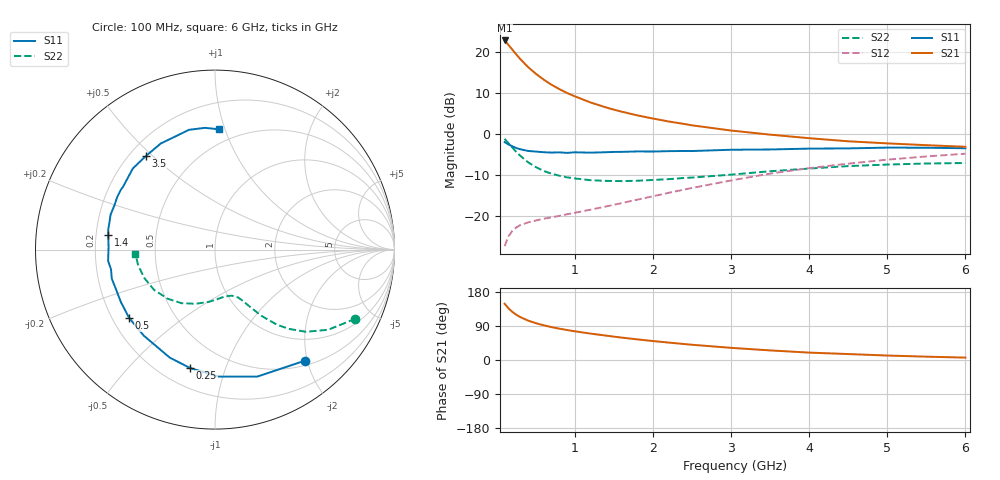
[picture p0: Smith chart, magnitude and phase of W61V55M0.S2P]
! SIEMENS Small Signal Semiconductors
! BFR193W
! Si NPN RF Bipolar Junction Transistor in SOT323
! VCE = 1.5 V  IC = 5 mA
! Common Emitter S-Parameters:  September  1992
# GHz  S  MA  R  50
!  f  S11  S21  S12  S22
! GHz  MAG  ANG  MAG  ANG  MAG  ANG  MAG  ANG
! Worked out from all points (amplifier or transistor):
!   28 points, 100 MHz to 6 GHz, reference 50 ohm
!   highest |S21| = 22.8 dB at 100 MHz (marker M1)
!   |S21| within 3 dB of that: start of sweep to 232 MHz
!   unconditionally stable (mu >= 1): 1.167 GHz to 2.661 GHz
!   at 300 MHz: K = 0.37, MSG = 20.2 dB, |S12| = -22.2 dB
!   at 1.5 GHz: K = 1.07, MAG = 10.0 dB, |S12| = -17.2 dB
!   at 6 GHz: K = 0.93, MSG = 0.8 dB, |S12| = -4.8 dB
!   S11 on the Smith chart (normalised r, x): 100 MHz: 0.58, -1.95; 250 MHz: 0.32, -0.76; 500 MHz: 0.27, -0.33; 1.4 GHz: 0.25, +0.06; 3.5 GHz: 0.26, +0.47; 6 GHz: 0.39, +0.96
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0.1  0.7958 -51.1  13.73 148.5  0.0432 64.7  0.8723 -26.2
0.15  0.7458 -71.6  12.08 136.3  0.0571 56.0  0.7727 -35.3
0.2  0.708 -88.4  10.59 126.7  0.0664 50.1  0.6832 -42.1
0.25  0.674 -101.9  9.265 119.3  0.0731 45.7  0.6037 -47.0
0.3  0.6526 -112.7  8.172 113.3  0.0778 42.8  0.5443 -50.4
0.4  0.6223 -129.7  6.524 104.0  0.084 40.0  0.4536 -54.8
0.5  0.6112 -141.5  5.399 97.2  0.0887 39.3  0.3954 -57.4
0.6  0.6003 -150.8  4.592 91.6  0.0931 39.6  0.3554 -59.6
0.7  0.5944 -158.0  3.973 86.8  0.0969 40.8  0.3292 -61.1
0.8  0.5974 -164.3  3.521 82.7  0.1009 42.1  0.3108 -62.8
0.9  0.5896 -169.3  3.151 79.1  0.1057 43.9  0.2969 -64.1
1  0.5989 -173.9  2.87 75.7  0.11 45.6  0.2881 -65.8
1.2  0.5932 178.5  2.418 69.7  0.1201 48.8  0.2742 -69.6
1.4  0.6003 172.3  2.102 64.3  0.1314 51.9  0.269 -73.6
1.8  0.6134 161.5  1.684 54.4  0.159 56.8  0.27 -82.4
2.2  0.6185 151.8  1.42 46.0  0.1923 59.5  0.2824 -91.2
2.5  0.6205 145.6  1.274 40.2  0.2205 60.3  0.2951 -97.8
3  0.6433 135.4  1.102 32.1  0.2722 59.7  0.3204 -109.6
3.5  0.6481 126.6  0.982 25.3  0.3299 57.0  0.3523 -122.1
4.5  0.6681 109.2  0.815 15.7  0.4356 48.4  0.407 -146.5
5.5  0.6807 94.7  0.731 8.8  0.5333 38.2  0.4373 -168.8
6  0.6704 88.0  0.699 6.3  0.5756 32.6  0.4439 -177.0
